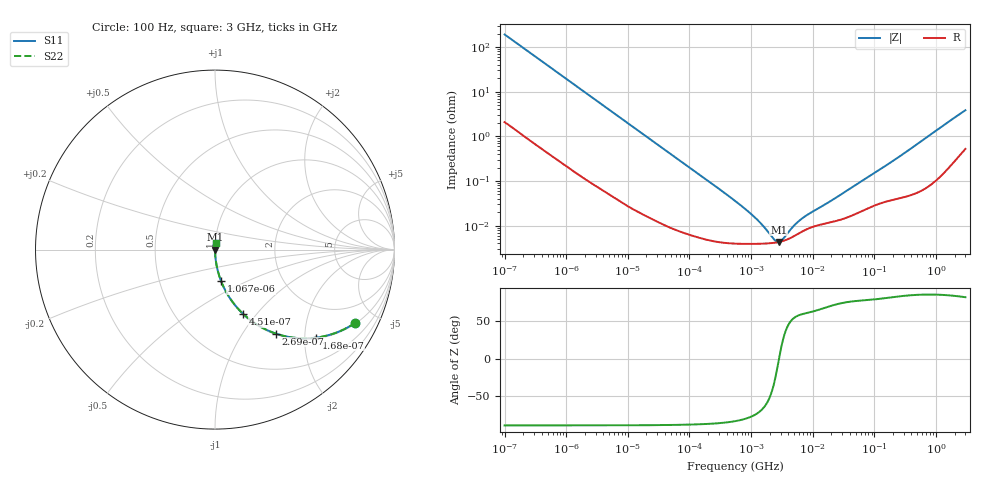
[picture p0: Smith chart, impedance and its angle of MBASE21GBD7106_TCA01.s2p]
! MBASE21GBD7106_TCA01  S-PARAMETER MODEL  ( Standard Model )
! Model Generated by TAIYO YUDEN Corporation (http://www.ty-top.com)
! Version 2.0
! TAIYO YUDEN Control No. 240328
! Copyright(c) 2022 TAIYO YUDEN CO.,LTD. All Rights Reserved.
! Product Description (link to TY-COMPAS)
! https://ds.yuden.co.jp/TYCOMPAS/or/detail?pn=MBASE21GBD7106KTCA01&u=M
! Products Name : Multilayer Ceramic Capacitors
! Characteristics :
!  Capacitance : 10 [uF] , Rated Voltage : 16 [V] , TCC : X7T
!  Case Size : 2.0 x 1.25 / 0.079 x 0.049 [mm/inch] , Thickness : 1.25 / 0.049 [mm/inch]
!  (Conditions: Temperature = 25 [degC] , DC Bias Voltage = 0 [V])
! External Node Assignments :
!  1  o---| |---o  2
! GND o---------o GND
! Frequency Range : 100Hz  -  3GHz  [ 401 STEP ]
# MHZ S RI R 50
! Freq[MHz].  S11 Real  S11 Imag  S21 Real  S21 Imag  S12 Real  S12 Imag  S22 Real  S22 Imag
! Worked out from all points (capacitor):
!   401 points, 100 Hz to 3 GHz, reference 50 ohm
!   read as one part in series: C = 8.33 uF near 109 Hz
!   lowest |Z| = 4.3 mohm at 2.811 MHz (marker M1)
!   series resonance near 2.838 MHz, so ESL is about 380 pH
!   S11 on the Smith chart (normalised r, x): 100 Hz: 1.04, -3.81; 168 Hz: 1.02, -2.28; 269 Hz: 1.02, -1.43; 451 Hz: 1.01, -0.85; 1.067 kHz: 1.00, -0.36; 3 GHz: 1.01, +0.08
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0.0001  0.7818 -0.4076  0.2182 0.4076  0.2182 0.4076  0.7818 -0.4076
0.000119  0.7189 -0.4441  0.2811 0.4441  0.2811 0.4441  0.7189 -0.4441
0.000168  0.5655 -0.4903  0.4345 0.4903  0.4345 0.4903  0.5655 -0.4903
0.000269  0.3392 -0.4681  0.6608 0.4681  0.6608 0.4681  0.3392 -0.4681
0.000451  0.1572 -0.3586  0.8428 0.3586  0.8428 0.3586  0.1572 -0.3586
0.000664  0.0805 -0.2666  0.9195 0.2666  0.9195 0.2666  0.0805 -0.2666
0.001067  0.0338 -0.1753  0.9662 0.1753  0.9662 0.1753  0.0338 -0.1753
0.001788  0.0129 -0.1073  0.9871 0.1073  0.9871 0.1073  0.0129 -0.1073
0.005476  0.00174 -0.0357  0.9983 0.0357  0.9983 0.0357  0.00174 -0.0357
0.031977  0.000156 -0.00622  0.9998 0.00622  0.9998 0.00622  0.000156 -0.00622
0.547723  3.97e-05 -0.000357  1 0.000357  1 0.000357  3.97e-05 -0.000357
0.918067  3.9e-05 -0.000198  1 0.000198  1 0.000198  3.9e-05 -0.000198
1.53882  3.94e-05 -9.35e-05  1 9.35e-05  1 9.35e-05  3.94e-05 -9.35e-05
1.677156  3.96e-05 -7.91e-05  1 7.91e-05  1 7.91e-05  3.96e-05 -7.91e-05
2.81117  4.29e-05 -1.33e-06  1 1.33e-06  1 1.33e-06  4.29e-05 -1.33e-06
4.91919  5.78e-05 8e-05  0.9999 -8e-05  0.9999 -8e-05  5.78e-05 8e-05
7.246509  7.78e-05 0.000136  0.9999 -0.000136  0.9999 -0.000136  7.78e-05 0.000136
9.794414  9.3e-05 0.000181  0.9999 -0.000181  0.9999 -0.000181  9.3e-05 0.000181
22.1892  0.000124 0.000377  0.9999 -0.000377  0.9999 -0.000377  0.000124 0.000377
175.1444  0.000367 0.00246  0.9996 -0.00246  0.9996 -0.00246  0.000367 0.00246
1950.712  0.00328 0.0253  0.9967 -0.0253  0.9967 -0.0253  0.00328 0.0253
3000  0.00661 0.0376  0.9934 -0.0376  0.9934 -0.0376  0.00661 0.0376
